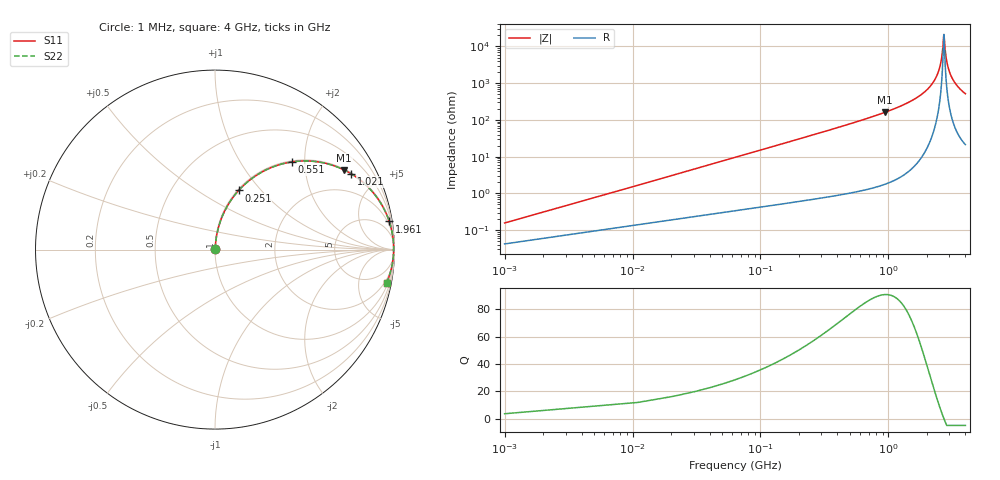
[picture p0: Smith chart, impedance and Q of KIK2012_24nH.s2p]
!version-2
!date-01.2022
!Series
# MHz S RI R 50
!Freq ReS11 ImS11 ReS21 ImS21 ReS12 ImS12 ReS22 ImS22
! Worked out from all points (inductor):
!   401 points, 1 MHz to 4 GHz, reference 50 ohm
!   read as one part in series: L = 24 nH near 21 MHz
!   highest Q = 90.9 at 941 MHz (marker M1), where L = 27.3 nH
!   self-resonance near 2.711 GHz
!   S11 on the Smith chart (normalised r, x): 1 MHz: 1.00, +0.00; 251 MHz: 1.01, +0.76; 551 MHz: 1.02, +1.73; 1.021 GHz: 1.04, +3.59; 1.961 GHz: 1, +12; 4 GHz: 1, -10
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1  0.000424 0.00151  0.9996 -0.00151  0.9996 -0.00151  0.000424 0.00151
31  0.00451 0.0464  0.9955 -0.0464  0.9955 -0.0464  0.00451 0.0464
61  0.0116 0.0907  0.9884 -0.0907  0.9884 -0.0907  0.0116 0.0907
131  0.042 0.1888  0.958 -0.1888  0.958 -0.1888  0.042 0.1888
251  0.1316 0.3293  0.8684 -0.3293  0.8684 -0.3293  0.1316 0.3293
551  0.4298 0.4888  0.5702 -0.4888  0.5702 -0.4888  0.4298 0.4888
671  0.5369 0.4928  0.4631 -0.4928  0.4631 -0.4928  0.5369 0.4928
941  0.7201 0.4435  0.2799 -0.4435  0.2799 -0.4435  0.7201 0.4435
1021  0.7603 0.4214  0.2397 -0.4214  0.2397 -0.4214  0.7603 0.4214
1341  0.8743 0.3255  0.1257 -0.3255  0.1257 -0.3255  0.8743 0.3255
1961  0.9709 0.1566  0.0291 -0.1566  0.0291 -0.1566  0.9709 0.1566
2001  0.9739 0.1471  0.0261 -0.1471  0.0261 -0.1471  0.9739 0.1471
2461  0.9934 0.0478  0.00655 -0.0478  0.00655 -0.0478  0.9934 0.0478
2591  0.995 0.023  0.00496 -0.023  0.00496 -0.023  0.995 0.023
2671  0.9954 0.00825  0.00462 -0.00825  0.00462 -0.00825  0.9954 0.00825
2701  0.9954 0.00285  0.00461 -0.00285  0.00461 -0.00285  0.9954 0.00285
2721  0.9954 -0.000721  0.00464 0.000721  0.00464 0.000721  0.9954 -0.000721
2811  0.9949 -0.0164  0.00507 0.0164  0.00507 0.0164  0.9949 -0.0164
2921  0.9938 -0.035  0.00625 0.035  0.00625 0.035  0.9938 -0.035
3091  0.9907 -0.0622  0.00929 0.0622  0.00929 0.0622  0.9907 -0.0622
3341  0.984 -0.0994  0.016 0.0994  0.016 0.0994  0.984 -0.0994
4000  0.9568 -0.1837  0.0432 0.1837  0.0432 0.1837  0.9568 -0.1837
